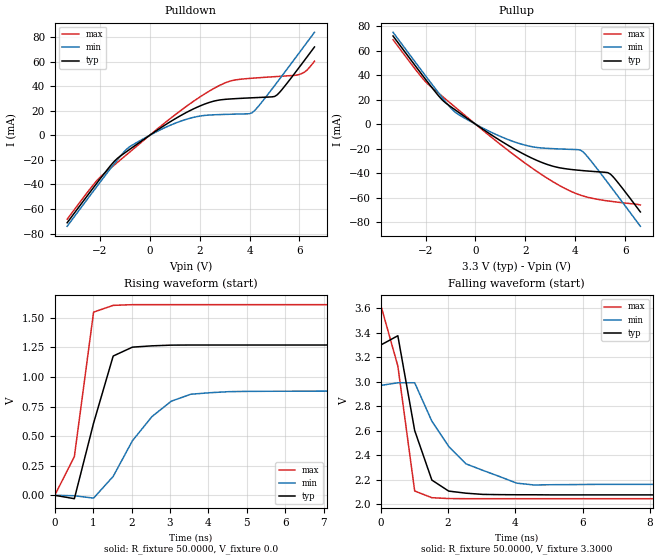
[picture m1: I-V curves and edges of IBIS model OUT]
| SEIKO EPSON CORPORATION
| IBIS file vg7050can1.ibs for VG7050CAN (up to 40MHz)
[IBIS ver] 3.2
[File name] vg7050can1.ibs
[File Rev] 1.0
[Date]  Apr 4 2014
[Source] This file originated at SEIKO EPSON Corporation.
[Notes]  1) Only OUT pin is reported in this file,
   VC pins as NC.
   2) Waveforms coming from the model may differ from
   those of actual ICs.
[Disclaimer]  This information is for modeling purposes only and
   is not guaranteed.
[Copyright] Copyright 2014, SEIKO EPSON Corporation,
   All Rights Reserved.
|   Component VG7050CAN
[Component] VG7050CAN
[Manufacturer] SEIKO EPSON
[Package]
| variable   typ   min   max
R_pkg   0.224   NA   NA
L_pkg   5.50n   NA   NA
C_pkg   1.45p   NA   NA
[Pin]  signal_name   model_name   R_pin   L_pin   C_pin
6   vdd   POWER   NA   NA   NA
5   nc   NC   NA   NA   NA
4   out   OUT   0.224   5.50n   1.45p
3   vss   GND   NA   NA   NA
2   oe   NC   NA   NA   NA
1   vc   NC   NA   NA   NA
| Models and submodels in the file (1): OUT (Output)
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|   Model OUT
[Model]  OUT
Model_type Output
Polarity   Inverting
C_comp   1pF   1pF   1pF
[Temperature Range]   25.0000   85.0000   -40.0000
[Voltage Range]   3.3000V   2.9700V   3.6300V
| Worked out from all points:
|   slope of the pulldown table from 0 to 0.495 V, typ, clamps not added: 72.7 ohm
|   slope of the pullup table from 0 to 0.495 V, typ, clamps not added: 72.4 ohm
|   rising waveform, R_fixture 50.0000, V_fixture 0.0: 20-80 % time 644ps typ, 1.13ns min, 402ps max; typ from 0 V to 1.27 V
|   falling waveform, R_fixture 50.0000, V_fixture 3.3000: 20-80 % time 647ps typ, 1.28ns min, 563ps max; typ from 3.3 V to 2.08 V
[Pulldown]
|Voltage   I(typ)   I(min)   I(max)
-3.3V     -71.2mA    -74.07mA   -68.31mA
-2.1V     -38.61mA   -41.37mA   -36.58mA
-1.4V     -20.89mA   -22.74mA   -23.94mA
-900mV    -12.91mA   -10.91mA   -15.38mA
800mV     10.76mA    8.001mA    13.26mA
2.1V      24.66mA    15.99mA    32.42mA
3.1V      29.47mA    17.13mA    43.38mA
4.1V      30.61mA    18.38mA    46.56mA
5.1V      32.91mA    43.13mA    47.95mA
6.1V      58.43mA    70.29mA    50.47mA
6.3V      63.85mA    75.76mA    53.15mA
6.6V      72.02mA    83.98mA    60.43mA
[Pullup]
|Voltage   I(typ)   I(min)   I(max)
-3.3V     71.85mA    74.86mA    68.81mA
-2V       36.56mA    39.44mA    34.62mA
-1.3V     19.16mA    20.89mA    22.19mA
-800mV    11.46mA    9.555mA    13.62mA
1.1V      -14.71mA   -10.88mA   -18.11mA
1.9V      -24.04mA   -16.63mA   -30.46mA
2.5V      -29.9mA    -19.1mA    -39.08mA
3.3V      -35.25mA   -20.14mA   -49.28mA
4.1V      -37.48mA   -20.77mA   -57.09mA
4.3V      -37.86mA   -22.47mA   -58.47mA
5.4V      -40.67mA   -50.53mA   -62.82mA
6.6V      -71.52mA   -83.22mA   -65.86mA
[Ramp]
| variable   typ   min   max
dV/dt_r  0.7620/0.6368n   0.5284/1.1236n   0.9666/0.4022n
dV/dt_f  0.7344/0.6399n   0.4848/1.2680n   0.9510/0.5592n
R_load = 50.0000
[Rising Waveform]
R_fixture= 50.0000
V_fixture= 0.0
V_fixture_min= 0.0
V_fixture_max= 0.0
|time   V(typ)   V(min)   V(max)
0s        0V         0V         0V
510ps     -28.46mV   -3.615mV   327.7mV
1.01ns    610.3mV    -23.7mV    1.548V
1.52ns    1.177V     159.9mV    1.605V
2.02ns    1.252V     460.9mV    1.611V
2.53ns    1.263V     665.6mV    1.611V
3.03ns    1.269V     795mV      1.611V
3.54ns    1.27V      854.1mV    1.611V
4.55ns    1.27V      876.2mV    1.611V
50ns      1.27V      880.7mV    1.611V
[Falling Waveform]
R_fixture= 50.0000
V_fixture= 3.3000
V_fixture_min= 2.9700
V_fixture_max= 3.6300
|time   V(typ)   V(min)   V(max)
0s        3.3V       2.97V      3.63V
510ps     3.376V     2.992V     3.129V
1.01ns    2.602V     2.992V     2.108V
1.52ns    2.197V     2.678V     2.053V
2.02ns    2.107V     2.472V     2.046V
2.53ns    2.09V      2.33V      2.045V
3.03ns    2.08V      2.277V     2.045V
4.04ns    2.077V     2.172V     2.045V
4.55ns    2.077V     2.157V     2.045V
50ns      2.076V     2.162V     2.045V
